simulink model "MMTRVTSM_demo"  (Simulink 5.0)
settings: Solver=ode45  StartTime=0.0  StopTime=100  RelTol=1e-3
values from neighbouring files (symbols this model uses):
  A = [ 1      (-1/b1)    [DRVTS1.m]    (also in DRVTS_M.m = DRVTS_A(l,n,d1,d3,h,m1,m3,ro,cp,ka); JRVTS_M.m = JRVTS_A(l,n,d12,d23,m1,ro1,cp1,alfa12); MATICA.M = matica_A(h,a,d,e,f); TRVTS1.m = [(1-Z12/b1)  (-Z23/b1))
  B = [(a1/b1*ts1(i))    [DRVTS1.m]    (also in DRVTS_M.m = DRVTS_B(l,n,d1,d3,h,m1,m3,ro,cp,ka,pom); JRVTS_M.m = JRVTS_B(l,n,d12,d23,m1,ro1,cp1,alfa12,pom); MATICA.M = matica_B(a,c,d,f); TRVTS1.m)
  C = DRVTS_C(n,vystup)    [DRVTS_M.m]    (also in JRVTS_M.m = JRVTS_C(n,vystup); MATICA.M = matica_C(a,g); matica_C.m = zeros(r,a))
  x0 = TS    [DRVTSS.m]    (also in DRVTS_M.m = ts'; JRVTSS.m = JRVTS1(t1,t3,l,n,d1,d3,m1,ro1,cp1,ka); JRVTS_M.m = ts'; KOLONA2.M = zeros(1,N+2))
undefined symbols (not defined in the file or in its folder): TT

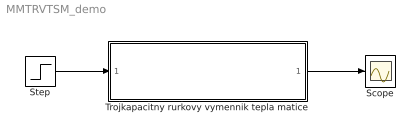
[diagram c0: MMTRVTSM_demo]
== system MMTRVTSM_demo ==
  Scope : Scope
  Step : Step  Time=0  Before=[75]  After=[75]  SampleTime=0
  Trojkapacitny rurkovy vymennik tepla matice : Subsystem  mask(TROJKAPACITNY RURKOVY VYMENNIK TEPLA - súprudový-matice){vst=[0 1], por=[0 0], teplota=[20 75], m=[1100/3600 400/3600], par1=[810 2.1e3 750], par3=[1000 4.2e3 1480], par2=[8930 385], par4=[25e-3 50e-3 1.5e-3], l=10, n=5, vystup=[0 0 0, 0 0 0, 1 0 0, 0 0 0, 1 0 1], mat=on}
      mask prompts: vst "Vstupné - riadiace velièiny   1-áno  0-nie    [T1 T3]"; por "Poruchové velièiny    1-áno  0-nie    [T1 T3]"; teplota "Vstupné teploty  [vnútorná vonkajšia] rúrka  [T1   T3]"; m "Vstupné hmotnostné toky   [vnútorná    vonkajšia]   rúrka   [m1  m3]"; par1 "Parametre média vo vnútornej rúrke  [hustota  cp  alfa]"; par3 "Parametre média vo vonkajšej rúrke    [hustota  cp  alfa]"; par2 "Parametre rúrky    [hustota  cp]"; par4 "Priemery rúrok   [vnútornej  vonkajšej  hrúbka steny]"; l "Dlžka výmenníka tepla"; n "Poèet úsekov pri diskretizácii"; vystup "Vektor sledovaných velièín    [ .. T(1,i)  T(2,i)  T(3,i) .. ]"; mat "Vypísanie matíc A,B,C,D"
      mask help: Trojkapacitný súprudový rúrkový výmenník tepla -matice - lineárny model možnos� vo¾by riadiacich velièín - teploty vstupujúcich médii.
      mask init:
      | pom=vst+por;
      | ro=[par1(1) par2(1) par3(1)];
      | cp=[par1(2) par2(2) par3(2)];
      | ka=[par1(3) par3(3)];
      | d1=par4(1);
      | d3=par4(2);
      | h=par4(3);
      | t1=teplota(1);
      | t3=teplota(2);
      | m1=m(1);
      | m3=m(2);
      | TRVTS_M;
      | if mat == 1
      | 	A,B,C
      | 	D = TRVTS_D(B,C)
      | end
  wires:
  Step/1 -> Trojkapacitny rurkovy vymennik tepla matice/1(In1)
  Trojkapacitny rurkovy vymennik tepla matice/1(Out1) -> Scope/1

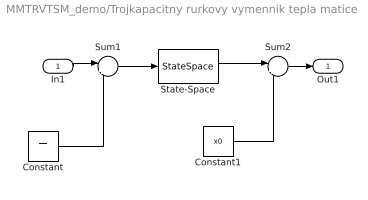
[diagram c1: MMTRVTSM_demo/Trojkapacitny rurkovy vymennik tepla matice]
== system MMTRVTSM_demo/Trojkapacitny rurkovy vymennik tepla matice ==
  In1 : Inport
  Constant : Constant  Value=TT
  Constant1 : Constant  Value=x0
  State-Space : StateSpace  A=A  B=B  C=C  D=D
  Sum1 : Sum  Inputs=|+-
  Sum2 : Sum  Inputs=|++
  Out1 : Outport
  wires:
  Sum1/1 -> State-Space/1
  State-Space/1 -> Sum2/1
  Constant/1 -> Sum1/2
  Constant1/1 -> Sum2/2
  In1/1 -> Sum1/1
  Sum2/1 -> Out1/1
